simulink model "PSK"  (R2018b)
settings: Solver=VariableStepAuto  StartTime=0.0  StopTime=20  FixedStep=1e-5  RelTol=1e-3
libraries: commdigbbndpm3 x2, commchan3 x1, commrandsrc3 x1, dspsrcs4 x1

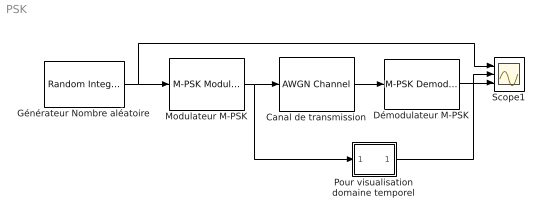
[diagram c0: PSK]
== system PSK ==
  Canal de transmission : commchan3/AWGN Channel  InputProcessing=Columns as channels (frame based)  seed=67  noiseMode="Signal to noise ratio  (SNR)"  EbNodB=10  EsNodB=10  SNRdB=30  bitsPerSym=1  Ps=1  Tsym=1  variance=1
  Démodulateur M-PSK : commdigbbndpm3/M-PSK Demodulator Baseband  M=8  OutType=Integer  DecType=Hard decision  VarSource=Dialog  Variance=1  Dec=Binary  Mapping=[0:7]  Ph=0  outDtype1=Inherit via internal rule  outDtype2=Inherit via internal rule  derotateFactorWordLen=16  derotateFactorDataTypeStr=Inherit: Same word length as input  derotateFactorLastDataTypeStr=Inherit: Same word length as input
  Générateur Nombre aléatoire : commrandsrc3/Random Integer Generator  SetSize=8  SeedSource=Auto  Seed=0  SampleTime=1  SamplesPerFrame=1  OutputDataType=double  SimulateUsing=Interpreted execution
  Modulateur M-PSK : commdigbbndpm3/M-PSK Modulator Baseband  M=8  InType=Integer  Enc=Binary  Mapping=[0:7]  Ph=0  outDtype=double  outWordLen=16  outUDDataType=sfix(16)  outFracLenMode=Best precision  outFracLen=15  outDataTypeStr=double  outLastDataTypeStr=double
  Pour visualisation domaine temporel : Subsystem
  Scope1 : Scope  NumInputPorts=3
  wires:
  Modulateur M-PSK/1 -> Canal de transmission/1, Pour visualisation domaine temporel/1(In1)
  Canal de transmission/1 -> Démodulateur M-PSK/1
  Générateur Nombre aléatoire/1 -> Scope1/1, Modulateur M-PSK/1
  Démodulateur M-PSK/1 -> Scope1/3
  Pour visualisation domaine temporel/1(Out1) -> Scope1/2

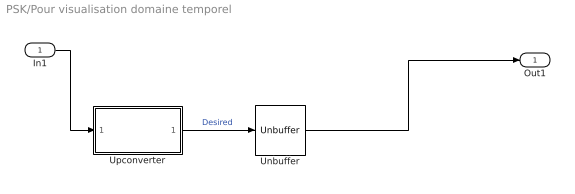
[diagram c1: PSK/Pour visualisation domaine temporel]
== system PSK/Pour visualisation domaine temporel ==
  In1 : Inport
  Unbuffer : Unbuffer
  Upconverter : Subsystem
  Out1 : Outport
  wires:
  Unbuffer/1 -> Out1/1
  Upconverter/1(Out) -> Unbuffer/1  "Desired"
  In1/1 -> Upconverter/1(In)

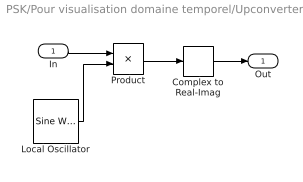
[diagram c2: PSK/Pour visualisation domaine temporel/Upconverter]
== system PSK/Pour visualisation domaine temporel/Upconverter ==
  In : Inport
  Complex to Real-Imag : ComplexToRealImag  Output=Real
  Local Oscillator : dspsrcs4/Sine Wave  Amplitude=1  Frequency=20  Phase=0  SampleMode=Discrete  OutComplex=Complex  CompMethod=Trigonometric fcn  TableSize=Speed  SampleTime=1/100000  SamplesPerFrame=100000  ResetState=Restart at time zero  OutputFrames=off  dataType=double  wordLen=16  udDataType=sfix(16)  fracBitsMode=Best precision  numFracBits=15  OutDataTypeStr=double  LastOutDataTypeStr=double
  Product : Product
  Out : Outport
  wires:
  Complex to Real-Imag/1 -> Out/1
  Product/1 -> Complex to Real-Imag/1
  Local Oscillator/1 -> Product/2
  In/1 -> Product/1
